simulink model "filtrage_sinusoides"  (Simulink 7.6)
settings: Solver=ode23t  StartTime=0.0  StopTime=0.16  RelTol=1e-3
InitFcn:
  | R=1;
  | L=0.01;
StopFcn:
  | close all
  | load Sinusoïdes_filtrage.mat
  | plot(x(1,:),x(2,:))
  | hold on
  | plot(x(1,:),x(3,:))
  | plot(x(1,:),x(4,:))
  | grid
  | title('Somme des 3 sinusoïdes, sinusoïde de 10 Hz et sortie du filtre')
  | xlabel('temps')
  | 
  | figure
  | 
  | close all
  | load fondamental.mat
  | plotyy(y(1,:),y(2,:),y(1,:),y(3,:))
  | grid
  | title('Amplitude et phase du fondamental  de 10 Hz')
  | xlabel('temps')
  | 
  | figure
  | 
  | close all
  | load RMS_x3.mat
  | plot(z(1,:),z(2,:))
  | grid
  | title('Valeur efficace de la sinusoïde x3 de 1 kHz')
  | xlabel('temps')
  | 
  | delete *.mat
libraries: powerlib x9, powerlib_extras x3

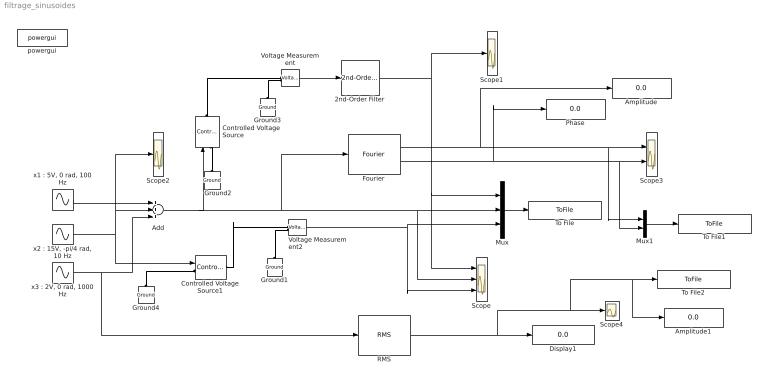
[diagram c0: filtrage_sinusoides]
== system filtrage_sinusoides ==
  2nd-Order Filter : powerlib_extras/Control  Blocks/2nd-Order Filter  DialogController=POWERSYS.PowerSysDialog  SystemSampleTime=-1  FilterType=Lowpass  Fo=15  Zeta=sqrt(2)/2  Initialize=off  Vac_Init=[1 45 60]  Vdc_Init=0  PlotResponse=on  param1=[1 200 1]
  Add : Sum  Inputs=+++
  Amplitude : Display
  Amplitude1 : Display
  Controlled Voltage Source : powerlib/Electrical Sources/Controlled Voltage Source  DialogController=POWERSYS.PowerSysDialog  SystemSampleTime=-1  Initialize=on  Source_Type=AC  Amplitude=0  Phase=0  Frequency=0  Measurements=None
  Controlled Voltage Source1 : powerlib/Electrical Sources/Controlled Voltage Source  DialogController=POWERSYS.PowerSysDialog  SystemSampleTime=-1  Initialize=on  Source_Type=AC  Amplitude=0  Phase=0  Frequency=0  Measurements=None
  Display1 : Display
  Fourier : powerlib_extras/Measurements/Fourier  DialogController=POWERSYS.PowerSysDialog  SystemSampleTime=-1  f1=10  n=1
  Ground{1..4} (4 alike) : powerlib/Elements/Ground  DialogController=POWERSYS.PowerSysDialog  PhysicalDomain=powersysdomain  SubClassName=unknown  LeftPortType=p1  RightPortType=p1  LConnTagsString=a
  Mux : Mux  Inputs=3
  Mux1 : Mux  Inputs=2
  Phase : Display
  RMS : powerlib_extras/Measurements/RMS  DialogController=POWERSYS.PowerSysDialog  SystemSampleTime=-1  f1=60
  Scope : Scope  NumInputPorts=3
  Scope1 : Scope
  Scope2 : Scope
  Scope3 : Scope  NumInputPorts=2
  Scope4 : Scope
  To File : ToFile  Filename=Sinusoïdes_filtrage  MatrixName=x
  To File1 : ToFile  Filename=fondamental  MatrixName=y
  To File2 : ToFile  Filename=RMS_x3  MatrixName=z
  Voltage Measurement : powerlib/Measurements/Voltage Measurement  DialogController=POWERSYS.PowerSysDialog  SystemSampleTime=-1  PhasorSimulation=off  OutputType=Complex  PSBequivalent=0
  Voltage Measurement2 : powerlib/Measurements/Voltage Measurement  DialogController=POWERSYS.PowerSysDialog  SystemSampleTime=-1  PhasorSimulation=off  OutputType=Complex  PSBequivalent=0
  powergui : powerlib/powergui  SystemSampleTime=-1  SimulationMode=Continuous  SampleTime=0  frequency=60  SPID=off  DisableSnubberDevices=off  DisableRonSwitches=off  DisableVfSwitches=off  SwTol=0  Interpol=off  frequencyindice=0  echomessages=off  HookPort=off  DisplayEquations=off  FunctionMessages=off  EnableUseOfTLC=off  x0status=blocks  RestoreLinks=warning  ResistiveCurrentMeasurement=off  Frange=[0:2:500]  Ylog=off  Xlog=on  ShowGrid=off  save=off  variable=ZData  structure=ScopeData1  ZoomFFT=off  StartTime=0.0  cycles=1  DisplayStyle=1  fundamental=10  FreqAxis=off  MaxFrequency=100  frequencyindicesteady=60  RmsSteady=1  display=off  Ts=0  methode=off
  "x1 : 5V, 0 rad, 100 Hz" : Sin  Amplitude=5  Frequency=2*pi*100  SampleTime=0
  "x2 : 15V, -pi/4 rad, 10 Hz" : Sin  Amplitude=15  Frequency=2*pi*10  Phase=-pi/4  SampleTime=0
  "x3 : 2V, 0 rad, 1000 Hz" : Sin  Amplitude=2  Frequency=2*pi*1e3  SampleTime=0
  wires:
  Add/1 -> Controlled Voltage Source/1, Fourier/1, Mux/2, Scope/2
  2nd-Order Filter/1 -> Scope1/1, Mux/1, Scope/1
  Mux/1 -> To File/1
  "x1 : 5V, 0 rad, 100 Hz"/1 -> Add/1
  "x2 : 15V, -pi/4 rad, 10 Hz"/1 -> Controlled Voltage Source1/1, Add/2, Scope2/1
  Voltage Measurement/1 -> 2nd-Order Filter/1
  "x3 : 2V, 0 rad, 1000 Hz"/1 -> Add/3, RMS/1
  Voltage Measurement2/1 -> Mux/3, Scope/3
  Fourier/1 -> Amplitude/1, Scope3/1, Mux1/1
  Fourier/2 -> Phase/1, Scope3/2, Mux1/2
  RMS/1 -> Display1/1, Scope4/1, To File2/1, Amplitude1/1
  Mux1/1 -> To File1/1
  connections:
  Ground2/LConn1 -- Controlled Voltage Source/LConn1
  Controlled Voltage Source/RConn1 -- Voltage Measurement/LConn1
  Ground3/LConn1 -- Voltage Measurement/LConn2
  Controlled Voltage Source1/RConn1 -- Voltage Measurement2/LConn1
  Ground1/LConn1 -- Voltage Measurement2/LConn2
  Ground4/LConn1 -- Controlled Voltage Source1/LConn1
